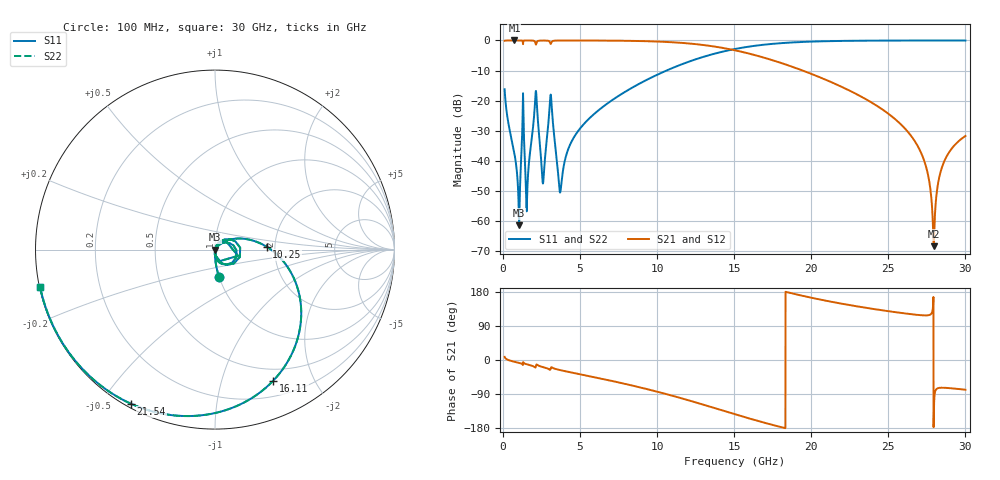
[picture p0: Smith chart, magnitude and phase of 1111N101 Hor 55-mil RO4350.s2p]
# GHz S MA R 50
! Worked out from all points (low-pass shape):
!   3201 points, 100 MHz to 30 GHz, reference 50 ohm
!   highest |S21| = -0.01 dB at 735.4 MHz (marker M1); lowest = -68.3 dB at 27.94 GHz (marker M2)
!   |S21| within 3 dB of the highest: start of sweep to 14.8 GHz
!   lowest |S11| = -61.3 dB at 1.044 GHz (marker M3), VSWR 1.00, Z = 50.1 - j0.00523 ohm
!   |S11| at or under -10 dB: start of sweep to 10.6 GHz
!   |S22| runs from -61.3 to 0.0 dB; largest |S21 - S12| = 0
!   S11 on the Smith chart (normalised r, x): 100 MHz: 1.00, -0.31; 10.25 GHz: 1.81, +0.06; 16.11 GHz: 0.36, -1.47; 21.54 GHz: 0.01, -0.59; 30 GHz: 0.00, -0.11
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0.1  0.1546 -81.7  0.9877 8.2  0.9877 8.2  0.1546 -81.7
0.735375  0.01334 -92.2  0.9993 -4.6  0.9993 -4.6  0.01334 -92.2
1.043719  0.0008567 -3.5  0.999 -7.6  0.999 -7.6  0.0008567 -3.5
1.286656  0.1123 23.8  0.908 -13.3  0.908 -13.3  0.1123 23.8
1.604344  0.005003 61.1  0.9983 -12.0  0.9983 -12.0  0.005003 61.1
2.108906  0.1324 14.0  0.8866 -19.5  0.8866 -19.5  0.1324 14.0
2.594781  0.004253 -9.4  0.9955 -18.8  0.9955 -18.8  0.004253 -9.4
3.127375  0.1048 -53.1  0.9108 -19.2  0.9108 -19.2  0.1048 -53.1
3.706688  0.003009 -14.8  0.9966 -26.7  0.9966 -26.7  0.003009 -14.8
5.089563  0.03699 48.8  0.9969 -38.4  0.9969 -38.4  0.03699 48.8
10.06978  0.2748 5.0  0.9575 -84.4  0.9575 -84.4  0.2748 5.0
10.24731  0.2883 3.2  0.9534 -86.2  0.9534 -86.2  0.2883 3.2
15.05  0.7211 -53.5  0.6858 -143.2  0.6858 -143.2  0.7211 -53.5
16.10584  0.7999 -66.2  0.5923 -155.8  0.5923 -155.8  0.7999 -66.2
20.03956  0.9572 -106.4  0.2763 164.0  0.2763 164.0  0.9572 -106.4
21.54391  0.9781 -118.6  0.1906 151.8  0.1906 151.8  0.9781 -118.6
25.01978  0.995 -142.0  0.06031 128.7  0.06031 128.7  0.995 -142.0
27.14081  0.9968 -153.8  0.01338 118.1  0.01338 118.1  0.9968 -153.8
27.58931  0.9969 -156.2  0.005662 118.1  0.005662 118.1  0.9969 -156.2
27.94438  0.9969 -158.0  0.0003858 -156.8  0.0003858 -156.8  0.9969 -158.0
28.57041  0.9969 -161.1  0.009078 -73.2  0.009078 -73.2  0.9969 -161.1
30  0.9966 -167.9  0.02599 -78.4  0.02599 -78.4  0.9966 -167.9
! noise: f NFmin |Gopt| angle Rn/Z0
0.1  0.0006913  0.7431  1.129  0.0005399
3.417  0.01874  0.6905  24.69  0.01126
6.743  0.01651  0.4331  45.43  0.0042
10.06  0.02424  0.4475  62.65  0.005624
13.39  0.0361  0.5209  78.32  0.008454
16.7  0.05735  0.6405  95.14  0.0145
20.03  0.1039  0.7789  114.1  0.02954
23.35  0.2383  0.8971  133.4  0.08041
26.67  1.187  0.9781  151.5  0.7566
30  1.031  0.9742  167.8  0.1052
